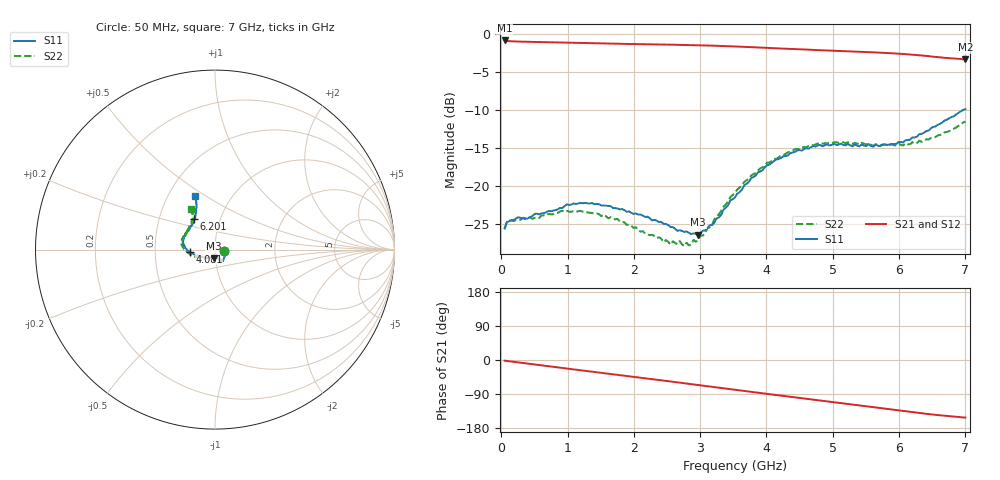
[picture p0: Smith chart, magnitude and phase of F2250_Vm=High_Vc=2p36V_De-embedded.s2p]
! Integrated Device Technology
! Corporate Headquarters
! 6024 Silver Creek Valley Road
! San Jose, CA 95138  USA
! Phone:  1-408-284-8200
! Toll Free:  1-800-223-1366
! Webpage:  http://www.idt.com/
! Timing and RF Division
! 515 Groton Road, Suite 102
! Westford, MA 01886-6024
! Device:  F2250
! Description: Voltage Variable RF Attenuator
! Frequency:  50.0 -  6000.00 MHz
! Package:  3x3 mm Thin QFN Plastic Package: 16 pin
! Ports:  2 RF, 3 DC
!  Pin  1  = GND
!  Pin  2  = NC
!  Pin  3  = RF1  = Port 1
!  Pin  4  = NC
!  Pin  5  = GND
!  Pin  6  = GND
!  Pin  7  = GND
!  Pin  8  = GND
!  Pin  9  = NC
!  Pin 10  = RF2  = Port 2
!  Pin 11  = NC
!  Pin 12  = GND
!  Pin 13  = GND
!  Pin 14  = VCNTRL
!  Pin 15  = VDD
!  Pin 16  = VMODE
! Vcntrl:  2.360 Volts
! Vmode:  +3.300 Volts
! Vdd:  +3.30  Volts
! Current:  1.316 mA
! Data:  The device was measured on a the F2250 evaluation board which has
!  individual transmission lines to the RF pins.  Data was collected
!  using a calibrated network analyzer.  The evaluation board was
!  de-embedded using a TRL calibration technique.
!  The reference plane is the edge of the package pin.
! Misc:  SN 10
!  Action Tracker AT0258
! Date Measured:  2014-11-26
! Date:  2015-10-15  MJV
! Note:
!  Integrated Device Technology supplies this data as a sample of measured
!  data at the package pin for this product.  Your particular data for this
!  product may vary.
!  Data was taken at 25 degrees C.
!  Integrated Device Technology reserves the right to change this data at anytime.
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# GHz S dB R 50
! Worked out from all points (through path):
!   201 points, 50 MHz to 7 GHz, reference 50 ohm
!   highest |S21| = -0.90 dB at 50 MHz (marker M1); lowest = -3.4 dB at 7 GHz (marker M2)
!   group delay of S21, straight-line fit = 61.2 ps
!   lowest |S11| = -26.4 dB at 2.969 GHz (marker M3), VSWR 1.10, Z = 49.2 - j4.67 ohm
!   |S11| at or under -10 dB: start of sweep to 6.973 GHz
!   |S22| runs from -27.9 to -11.6 dB; largest |S21 - S12| = 0.002
!   S11 on the Smith chart (normalised r, x): 50 MHz: 1.11, -0.02; 4.081 GHz: 0.75, -0.02; 6.201 GHz: 0.75, +0.27; 7 GHz: 0.68, +0.45
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0.05  -25.55 -10.6  -0.90 -1.8  -0.90 -1.8  -25.72 -10.8
0.1195  -24.65 -10.1  -0.99 -3.2  -0.99 -3.2  -24.59 -8.8
0.57125  -23.75 -31.1  -1.11 -13.3  -1.11 -13.3  -24.23 -31.2
0.91875  -22.93 -49.8  -1.18 -21.0  -1.18 -21.1  -23.27 -50.8
1.2315  -22.30 -57.6  -1.24 -27.9  -1.24 -27.9  -23.40 -61.3
1.75275  -22.96 -64.5  -1.33 -39.1  -1.33 -39.1  -24.33 -67.7
2.37825  -24.77 -64.2  -1.43 -52.8  -1.43 -52.8  -26.76 -66.9
2.552  -25.42 -69.1  -1.45 -56.7  -1.45 -56.7  -27.73 -73.4
2.691  -25.83 -77.1  -1.48 -59.8  -1.48 -59.8  -27.25 -81.0
2.7605  -26.06 -79.3  -1.49 -61.3  -1.49 -61.3  -27.93 -85.5
2.969  -26.42 -97.2  -1.53 -66.0  -1.53 -66.0  -27.17 -104.9
3.1775  -25.17 -120.3  -1.58 -70.7  -1.58 -70.7  -25.16 -126.7
3.525  -21.54 -152.3  -1.69 -78.5  -1.69 -78.6  -20.93 -148.7
3.76825  -18.98 -164.5  -1.78 -84.0  -1.78 -84.1  -18.66 -159.6
4.081  -16.97 -175.5  -1.91 -91.0  -1.90 -91.0  -16.70 -171.4
4.4285  -15.55 176.2  -2.04 -98.6  -2.04 -98.7  -15.18 178.7
4.7065  -14.78 169.2  -2.14 -104.8  -2.14 -104.8  -14.67 173.0
5.054  -14.62 161.1  -2.27 -112.5  -2.26 -112.5  -14.27 165.9
5.85325  -14.59 135.2  -2.57 -130.0  -2.56 -130.1  -14.68 147.2
6.20075  -13.64 123.7  -2.77 -137.7  -2.78 -137.8  -14.26 138.2
6.54825  -12.20 115.7  -3.05 -144.7  -3.05 -144.9  -13.59 126.9
7  -9.92 110.8  -3.37 -152.1  -3.38 -152.2  -11.55 120.6
